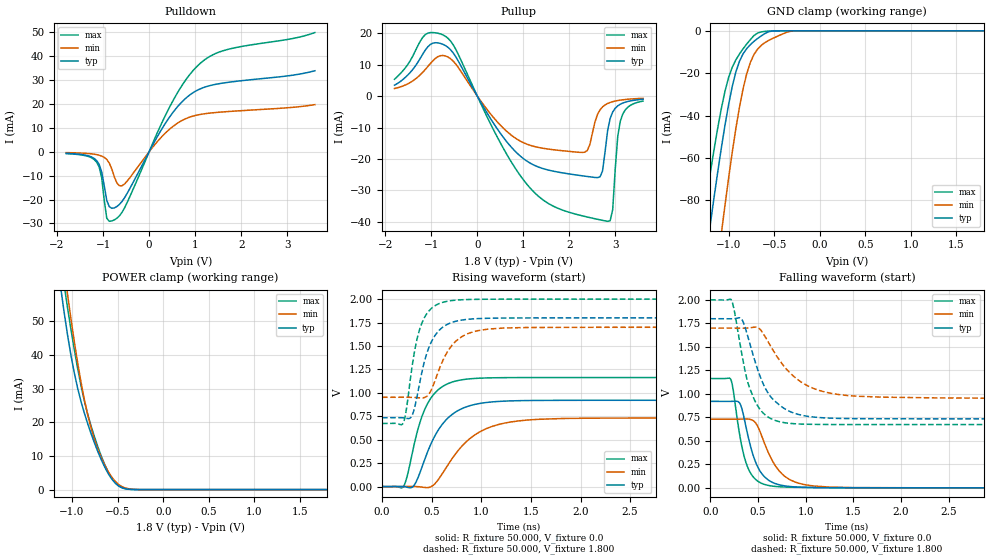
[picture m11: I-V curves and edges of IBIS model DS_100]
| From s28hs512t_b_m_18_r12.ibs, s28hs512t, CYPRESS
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|   Model DS_100
[Model] DS_100
Model_type 3-state
Polarity   Non-Inverting
Enable   Active-High
Vmeas =  0.900V
Cref =  15.000pF
C_comp   5.334pF   5.23pF   5.767pF
[Temperature Range]   25.000   0.125k   -40.000
[Voltage Range]   1.800V   1.700V   2.000V
[Pullup Reference]   1.800V   1.700V   2.000V
[Pulldown Reference]   0.0V   0.0V   0.0V
[POWER Clamp Reference]   1.800V   1.700V   2.000V
[GND Clamp Reference]   0.0V   0.0V   0.0V
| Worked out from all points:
|   slope of the pulldown table from 0 to 0.27 V, typ, clamps not added: 28.8 ohm
|   slope of the pullup table from 0 to 0.27 V, typ, clamps not added: 39.9 ohm
|   GND clamp passes 1 mA (typ) near -0.59 V on its own axis
|   POWER clamp passes 1 mA (typ) near -0.48 V on its own axis
|   rising waveform, R_fixture 50.000, V_fixture 0.0: 20-80 % time 275ps typ, 374ps min, 204ps max; typ from 0 V to 0.921 V
|   rising waveform, R_fixture 50.000, V_fixture 1.800: 20-80 % time 169ps typ, 219ps min, 138ps max; typ from 0.734 V to 1.8 V
|   falling waveform, R_fixture 50.000, V_fixture 0.0: 20-80 % time 162ps typ, 227ps min, 131ps max; typ from 0.921 V to 0 V
|   falling waveform, R_fixture 50.000, V_fixture 1.800: 20-80 % time 252ps typ, 383ps min, 184ps max; typ from 1.8 V to 0.734 V
[Pulldown]
|Voltage   I(typ)   I(min)   I(max)
-1.8V     -643.1uA   -344uA     -754.9uA
-1.14V    -3.675mA   -1.183mA   -4.301mA
-1.03V    -8.433mA   -1.79mA    -10.89mA
-920mV    -20.33mA   -3.208mA   -27.82mA
-755mV    -23.48mA   -10.51mA   -28.49mA
-645mV    -22.02mA   -14.2mA    -26.81mA
-535mV    -19.28mA   -13.5mA    -23.52mA
400mV     13.3mA     8.7mA      17.03mA
730mV     21.23mA    13.26mA    28.24mA
1.06V     25.89mA    15.44mA    36.14mA
1.665V    28.94mA    16.78mA    42.62mA
3.6V      33.92mA    19.74mA    49.9mA
[Pullup]
|Voltage   I(typ)   I(min)   I(max)
-1.8V     3.504mA    2.428mA    5.389mA
-1.13V    14.72mA    8.522mA    19.65mA
-690mV    16.11mA    12.81mA    19.08mA
520mV     -12.26mA   -9.553mA   -15.44mA
1.18V     -21.63mA   -15.83mA   -29.85mA
2.335V    -25.52mA   -17.87mA   -38.37mA
2.665V    -25.75mA   -4.35mA    -39.45mA
2.83V     -10.96mA   -2.336mA   -39.92mA
2.94V     -5.052mA   -1.754mA   -36.19mA
3.05V     -3.086mA   -1.397mA   -12.74mA
3.105V    -2.563mA   -1.266mA   -8.003mA
3.6V      -983.6uA   -680uA     -1.572mA
[GND_clamp]
|Voltage   I(typ)   I(min)   I(max)
-1.8V     -294mA     -373mA     -247.3mA
-1.28V    -116.8mA   -168.5mA   -89.46mA
-1.2V     -91.34mA   -138.7mA   -67.04mA
-1.08V    -55.6mA    -96.11mA   -36.91mA
-1.04V    -44.83mA   -82.66mA   -28.74mA
-1V       -34.98mA   -69.76mA   -22.14mA
-920mV    -19.48mA   -46.23mA   -13.73mA
-800mV    -8.377mA   -20.18mA   -6.205mA
-680mV    -3.579mA   -8.59mA    -1.029mA
-560mV    -408.3uA   -4.544mA   -113.8uA
-280mV    -162.8nA   -73.51uA   -82.13nA
1.8V      272.8pA    325nA      188.3pA
[POWER_clamp]
|Voltage   I(typ)   I(min)   I(max)
-1.8V     236.7mA    239.1mA    251.1mA
-1.123V   59.68mA    73.25mA    67.66mA
-1.086V   52.46mA    65.42mA    60.6mA
-1.049V   45.83mA    57.89mA    53.9mA
-938mV    30.03mA    37.57mA    35.87mA
-864mV    22.62mA    26.6mA     26.18mA
-790mV    16.52mA    18.14mA    18.76mA
-716mV    11.21mA    11.92mA    12.63mA
-642mV    6.708mA    7.258mA    7.47mA
-494mV    1.178mA    1.619mA    1.205mA
-272mV    6.291uA    28.11uA    4.439uA
1.8V      0A         0A         0A
[Ramp]
| variable   typ   min   max
dV/dt_r   0.552/0.275n   0.438/0.373n   0.698/0.204n
dV/dt_f   0.639/0.252n   0.448/0.383n   0.796/0.184n
R_load = 50.000
[Rising Waveform]
R_fixture= 50.000
V_fixture= 0.0
V_fixture_min= 0.0
V_fixture_max= 0.0
|time   V(typ)   V(min)   V(max)
0s        3.15uV     4.457uV    4.885uV
209ps     1.001mV    571.7uV    -7.246mV
312ps     568.8uV    1.524mV    394.9mV
403ps     209.5mV    -5.639mV   751.7mV
491ps     450.6mV    -2.272mV   942.1mV
617ps     677.9mV    153.4mV    1.073V
797ps     828.2mV    422.7mV    1.138V
1.107ns   903.3mV    641.2mV    1.161V
1.568ns   919.2mV    717.4mV    1.163V
6ns       920.5mV    730.8mV    1.164V
[Rising Waveform]
R_fixture= 50.000
V_fixture= 1.800
V_fixture_min= 1.700
V_fixture_max= 2.000
|time   V(typ)   V(min)   V(max)
0s        734.5mV    952.8mV    673.4mV
215ps     733.3mV    953.4mV    681.2mV
296ps     745.7mV    952.2mV    1.229V
352ps     957.6mV    948.9mV    1.572V
418ps     1.297V     948.2mV    1.784V
522ps     1.593V     1.098V     1.922V
652ps     1.728V     1.427V     1.976V
873ps     1.786V     1.635V     1.996V
1.223ns   1.798V     1.691V     1.999V
6ns       1.8V       1.7V       2V
[Falling Waveform]
R_fixture= 50.000
V_fixture= 0.0
V_fixture_min= 0.0
V_fixture_max= 0.0
|time   V(typ)   V(min)   V(max)
0s        920.6mV    730.7mV    1.164V
216ps     920.4mV    730.4mV    1.151V
305ps     906.1mV    731.1mV    584.3mV
360ps     715mV      732.4mV    315.1mV
411ps     485.4mV    729.9mV    177.1mV
486ps     246.8mV    674.7mV    80.13mV
604ps     85.98mV    385.5mV    26.85mV
784ps     20.71mV    120.2mV    8.821mV
1.094ns   3.399mV    18.88mV    3.314mV
6ns       2.729uV    19.31uV    -1.586uV
[Falling Waveform]
R_fixture= 50.000
V_fixture= 1.800
V_fixture_min= 1.700
V_fixture_max= 2.000
|time   V(typ)   V(min)   V(max)
0s        1.8V       1.7V       2V
224ps     1.799V     1.7V       1.993V
325ps     1.799V     1.699V     1.454V
391ps     1.618V     1.701V     1.13V
476ps     1.323V     1.711V     908.3mV
583ps     1.048V     1.594V     770.1mV
723ps     883.4mV    1.361V     704.3mV
993ps     765.9mV    1.101V     677.3mV
1.433ns   737.5mV    982.9mV    673.6mV
6ns       734.5mV    952.8mV    673.4mV
